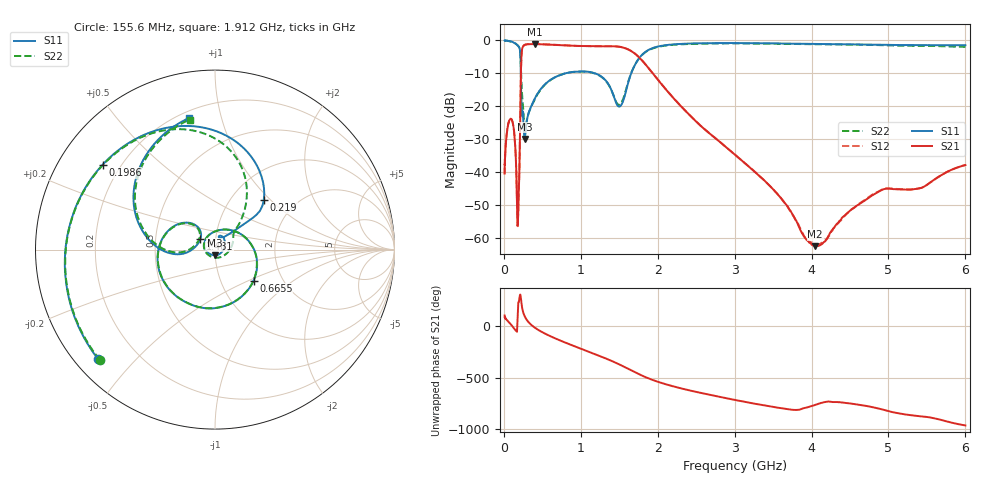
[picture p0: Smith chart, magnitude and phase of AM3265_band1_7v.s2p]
!Agilent Technologies,E8364B,MY43040894,A.07.50.67
!Agilent E8364B: A.07.50.67
!Date: Friday, May 09, 2025 07:17:05
!Correction: S11(Full 2 Port(1,2))
!S21(Full 2 Port(1,2))
!S12(Full 2 Port(1,2))
!S22(Full 2 Port(1,2))
!S2P File: Measurements: S11, S21, S12, S22:Log Frequency Sweep
# Hz S  dB  R 50
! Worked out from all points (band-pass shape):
!   3201 points, 10 MHz to 6 GHz, reference 50 ohm
!   highest |S21| = -1.11 dB at 400.5 MHz (marker M1); lowest = -62.6 dB at 4.047 GHz (marker M2)
!   |S21| within 3 dB of the highest: 230.7 MHz to 1.709 GHz (1.478 GHz wide, 152 % of centre)
!   lowest |S11| = -30.0 dB at 271.2 MHz (marker M3), VSWR 1.07, Z = 49.8 - j3.16 ohm
!   |S11| at or under -10 dB: 220.1 MHz to 800.4 MHz (580.3 MHz wide, 114 % of centre); 1.185 GHz to 1.656 GHz (470.7 MHz wide, 33.1 % of centre)
!   |S22| runs from -27.0 to -0.1 dB; largest |S21 - S12| = 0.0063
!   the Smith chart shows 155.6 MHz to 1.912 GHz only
!   S11 on the Smith chart (normalised r, x): 155.6 MHz: 0.07, -0.39; 198.6 MHz: 0.13, +0.33; 219 MHz: 1.40, +0.91; 665.5 MHz: 1.43, -0.54; 1.481 GHz: 0.84, +0.10; 1.912 GHz: 0.24, +0.79
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1e7  -0.05 -7.3  -40.28 105.7  -40.84 66.7  -0.10 -7.3
2.908064e7  -0.06 -21.1  -30.43 70.3  -30.39 69.6  -0.07 -21.1
8.439949e7  -0.25 -63.7  -23.87 24.9  -23.84 24.8  -0.28 -63.9
1.555967e8  -1.00 -137.1  -35.70 -41.6  -35.64 -41.1  -1.03 -136.3
1.796838e8  -1.51 -174.5  -56.11 90.3  -56.38 153.9  -1.50 -172.3
1.985718e8  -2.11 142.9  -42.91 -105.5  -42.96 -104.7  -2.05 148.3
2.19007e8  -8.21 45.6  -13.38 -70.5  -13.36 -70.5  -6.24 72.7
2.44949e8  -21.55 61.5  -2.06 155.2  -2.03 155.2  -18.62 29.9
2.712392e8  -29.97 -91.7  -1.36 97.8  -1.32 97.8  -26.82 -88.3
4.005401e8  -17.76 59.4  -1.11 -11.6  -1.08 -11.6  -17.90 61.7
6.65521e8  -11.18 -38.8  -1.35 -116.8  -1.32 -116.8  -11.20 -39.0
7.123273e8  -10.70 -52.2  -1.41 -131.8  -1.37 -131.8  -10.71 -52.6
1.146317e9  -9.74 -168.9  -1.78 100.0  -1.76 100.0  -9.80 -169.8
1.480576e9  -19.88 143.0  -1.86 -4.3  -1.83 -4.4  -19.41 144.7
1.912303e9  -2.53 101.3  -9.32 -157.0  -9.30 -157.0  -2.64 101.1
2.067357e9  -1.56 62.8  -13.81 163.3  -13.78 163.3  -1.68 63.2
2.450248e9  -0.92 -10.2  -23.52 88.5  -23.48 88.7  -1.05 -9.5
2.962692e9  -0.79 -89.2  -33.94 7.8  -33.92 7.9  -0.90 -89.4
3.511406e9  -0.90 -165.5  -45.58 -67.6  -45.55 -68.2  -1.00 -167.3
4.046889e9  -1.06 124.2  -62.58 -46.9  -62.21 -52.2  -1.17 121.8
5.002045e9  -1.35 4.3  -45.06 -108.8  -44.96 -109.0  -1.53 4.8
6e9  -1.44 -115.2  -37.91 112.8  -37.90 112.7  -1.95 -111.0
